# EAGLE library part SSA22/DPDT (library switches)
SW SLIDE DPDT 2POS SSA SER 30V
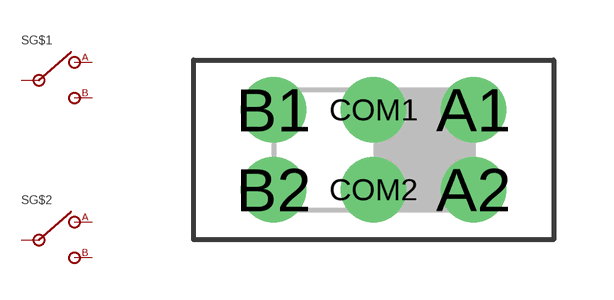
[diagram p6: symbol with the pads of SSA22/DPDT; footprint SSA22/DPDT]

Designator prefix S; gates G$1=SPDT G$2=SPDT

## SSA22/DPDT (DIGIKEY: 450-1604-ND; MOUSER: 506-SSA22; NEWARK: 50F5561)  [SSA22/DPDT]
A1  G$1:1
A2  G$2:1
B1  G$1:3
B2  G$2:3
COM1  G$1:2
COM2  G$2:2

## Footprint SSA22/DPDT (pad centres in mm)
drill 1.092: A1 2.5,1; A2 2.5,-1; B1 -2.5,1; B2 -2.5,-1; COM1 0,1; COM2 0,-1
